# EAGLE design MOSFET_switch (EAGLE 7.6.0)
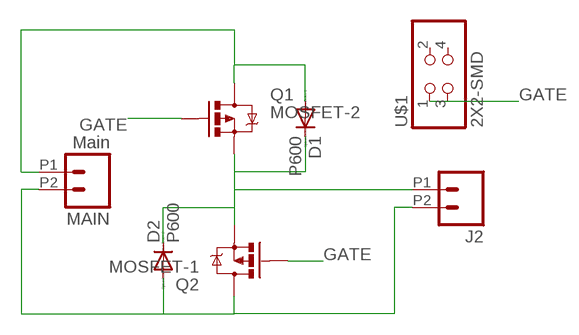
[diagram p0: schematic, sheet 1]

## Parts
D1  P600  [P6-15]
D2  P600  [P6-15]
J2  M022.54MM_SCREWTERM  [1X02_2.54_SCREWTERM]
MAIN  Main  M022.54MM_SCREWTERM  [1X02_2.54_SCREWTERM]
Q1  MOSFET-2  MOSFET-PCHANNELFQP27P06  [TO220V]
Q2  MOSFET-1  MOSFET-PCHANNELFQP27P06  [TO220V]
U$1  2X2-SMD  PINHD-2X2-SMD  [2X02SMD]

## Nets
GATE: Q1.1(G) Q2.1(G) U$1.1 U$1.3
N$1: D1.C D2.C J2.P1 Q1.3(S) Q2.3(S)
N$2: D2.A J2.P2 MAIN.P2 Q2.2(D)
N$5: D1.A MAIN.P1 Q1.2(D)
Unconnected: U$1.2 U$1.4

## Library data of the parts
D1 D2 = diode:P600: DIODE
J2 MAIN = SparkFun-Connectors:M02: Standard 2-pin 0.1" header. Use with
Q1 Q2 = SparkFun-DiscreteSemi:MOSFET-PCHANNEL: Generic PMOSFET IRLML2244 - TRANS-11153 (SOT-23 -20V -4.3A) (1.Gate 2.Source 3.Drain) FQP27P06 - COM-10349 (TO-220 -60V -27A) (1.Gate 2.Source 3.Drain)
U$1 = fab:PINHD-2X2-SMD

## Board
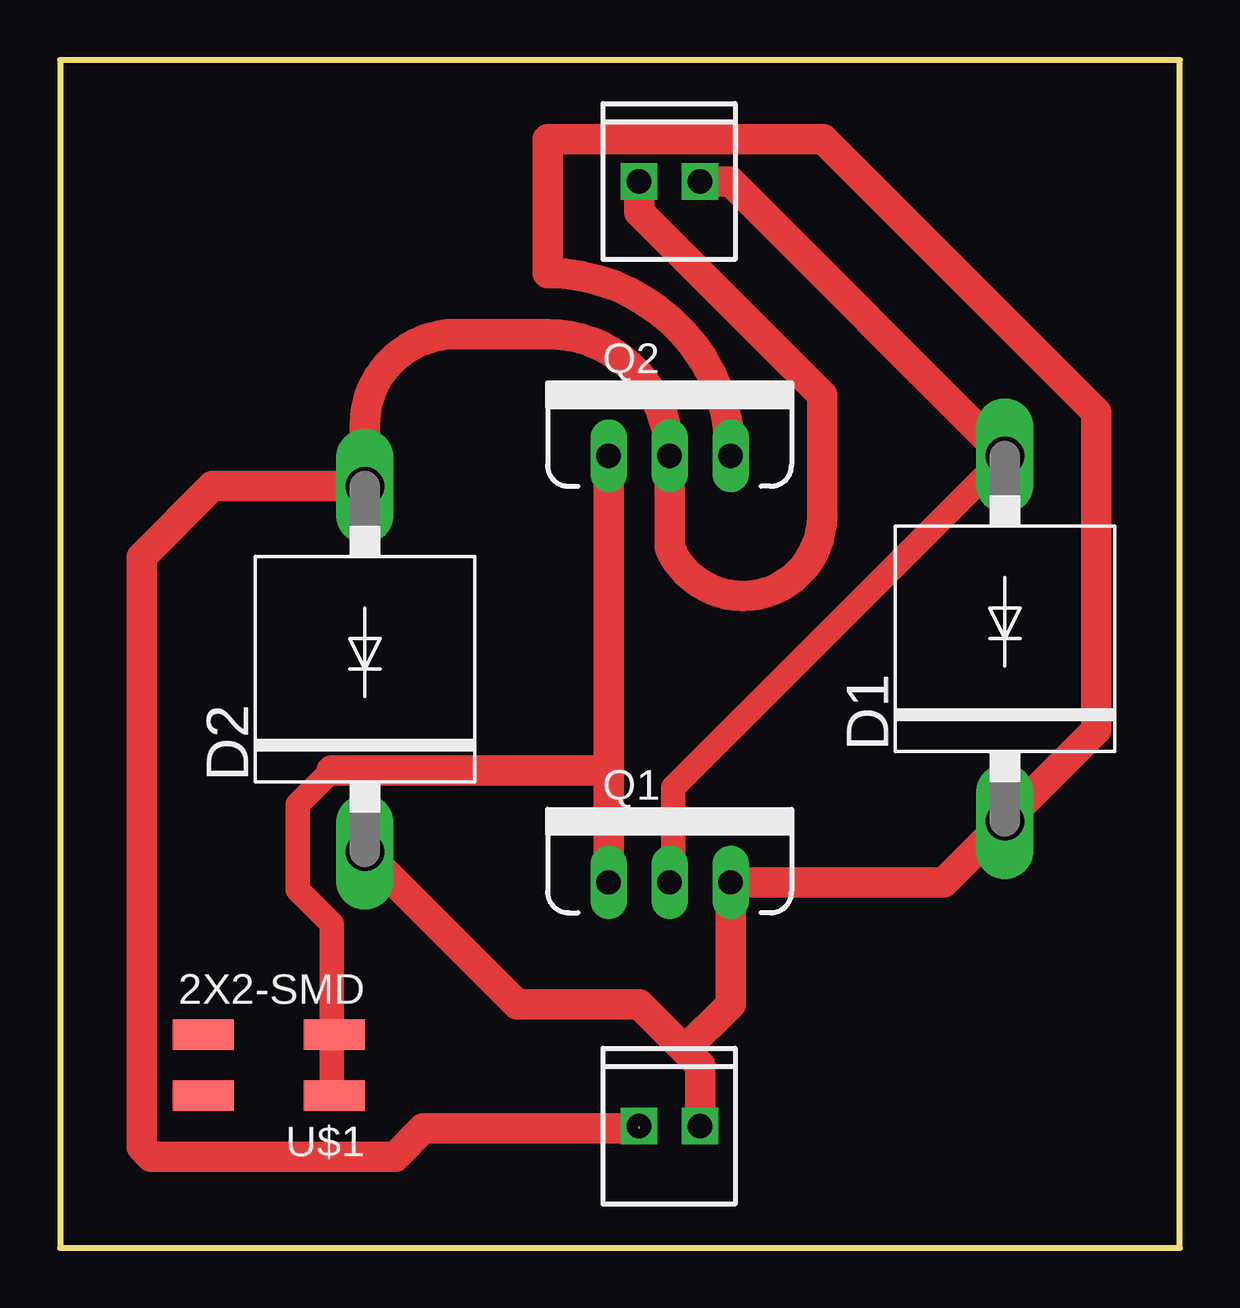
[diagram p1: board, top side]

Size 46.66 x 49.52 mm. Coordinates in mm from the lower left corner, seen from the top.
Outline: 0,0 46.66,0 46.66,49.52 0,49.52 0,0
Copper layers (1*16): Top 0.035mm / dielectric 1.5mm / Bottom 0.035mm
Design rules "default *": minimum track width 40mil, minimum drill 24mil, track to track 16mil, track to pad 16mil, pad to pad 8mil, via to via 8mil, smd to smd 8mil, copper to edge 40mil, drill to drill 16mil, minimum pad ring 10mil, minimum via ring 8mil, stop-mask expansion 4mil, vias tented up to drill 0mil, thermal gap 10mil

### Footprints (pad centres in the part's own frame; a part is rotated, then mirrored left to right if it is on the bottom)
P6-15 = drill 1.6 long: A 7.62,0; C -7.62,0
1X02_2.54_SCREWTERM = drill 1.016 square: P1 2.54,0; P2 0,0
TO220V = drill 1.016 long: 1 -2.54,0; 2 0,0; 3 2.54,0
2X02SMD = smd 2.54 x 1.27: 1 -2.54,1.27; 2 2.92,1.27; 3 -2.54,-1.27; 4 2.92,-1.27

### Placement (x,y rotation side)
D1  39.37,25.4 90 top
D2  12.7,24.13 90 top
J2  24.13,5.08 0 top
MAIN  24.13,44.45 0 top
Q1  25.4,15.24 0 top
Q2  25.4,33.02 0 top
U$1  8.89,7.62 180 top

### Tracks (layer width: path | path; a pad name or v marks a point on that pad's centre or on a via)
GATE
  Top 1.016: U$1.1 11.33,6.4 11.33,8.53 U$1.3 11.33,9.25 11.33,13.51 9.91,14.94 9.91,18.49 11.33,19.91
  Top 1.27: 22.86,19.91 11.33,19.91 | Q2.1 22.86,19.91 | Q1.1 22.86,19.91
N$1
  Top 1.27: Q2.3 arc90 20.32,40.64 20.32,46.23 31.8,46.23 43.18,34.85 43.18,21.59 D1.C 36.83,15.24 Q1.3 27.94,10.16 26.04,8.26 | D2.C 19.05,10.16 24.13,10.16 26.04,8.26 | J2.P1 26.67,7.62 26.04,8.26
N$2  (1 unrouted)
  Top 1.27: MAIN.P2 24.13,43.18 31.75,35.56 31.75,30.48 arc-157 25.4,29.21 Q2.2 arc90 20.32,38.1 16.51,38.1 arc90 12.7,34.29 D2.A 6.35,31.75 3.4,28.8 3.4,4.22 3.81,3.81 13.97,3.81 15.14,4.98 24.13,4.98
N$5
  Top 1.016: D1.A 25.55,19.2 25.55,15.65 Q1.2
  Top 1.27: MAIN.P1 27.94,44.45 D1.A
